FUNCTION_BLOCK "fb_517_alarm"
TITLE =Alarm-Modul (control buzzer and collective lamp)
//version!date    !author !change_segm!change_description
//-------+--------+-------+-----------+-------------------------------
// 1.0   !12.01.00!Kahle  ! ---       ! 1st version
// 1.1   !09.05.00!Kahle  ! 2         ! memo value DBD7 was wrong ->DBD17
AUTHOR : Kahle
FAMILY : PMA71
NAME : Alarm
VERSION : 1.1


VAR_INPUT
  IN_quittHorn : BOOL ;
  IN_acknowl : BOOL ;
  IN_flash : BOOL ;
END_VAR
VAR_OUTPUT
  OUT_Horn : BOOL ;
  OUT_lamp : BOOL ;
  OUT_alarm : BOOL ;
END_VAR
VAR
  Mask : ARRAY  [1 .. 5 ] OF DWORD ;
  Mask_2 : WORD ;
  memo : ARRAY  [1 .. 5 ] OF DWORD ;
  memo_2 : WORD ;
  horn_memo : BOOL ;
  alarm_memo : BOOL ;
END_VAR
VAR_TEMP
  relAlarm : ARRAY  [1 .. 5 ] OF DWORD ;
  relAlarm_2 : WORD ;
  alarmAvail : ARRAY  [1 .. 6 ] OF BOOL ;
END_VAR
BEGIN
NETWORK
TITLE =Geneate a collective alarm for alarm byte 1..4

      L     DB101.DBD   13;
      L     #Mask[1]; //release mask
      UD    ; //released alarms
      T     #relAlarm[1];
      L     #memo[1];
      XOD   ; //changed alarms
      L     #relAlarm[1];
      UD    ; //new alarms

      L     0;
      <>D   ; //if exist new alarms, set horn and flash lamp
      S     #horn_memo;
      S     #alarm_memo;
      L     DB101.DBD   13;
      T     #memo[1]; //store the actual alarms

      L     0;
      <>D   ;
      =     #alarmAvail[1]; //at least an alarm

NETWORK
TITLE =Geneate a collective alarm for alarm byte 5..8

      L     DB101.DBD   17;
      L     #Mask[2]; //release mask
      UD    ; //released alarms
      T     #relAlarm[2];
      L     #memo[2];
      XOD   ; //changed alarms
      L     #relAlarm[2];
      UD    ; //new alarms

      L     0;
      <>D   ; //if exist new alarms, set horn and flash lamp
      S     #horn_memo;
      S     #alarm_memo;
      L     DB101.DBD   17;
      T     #memo[2]; //store the actual alarms

      L     0;
      <>D   ;
      =     #alarmAvail[2]; //at least an alarm

NETWORK
TITLE =Geneate a collective alarm for alarm byte 9..12

      L     DB101.DBD   21;
      L     #Mask[3]; //release mask
      UD    ; //released alarms
      T     #relAlarm[3];
      L     #memo[3];
      XOD   ; //changed alarms
      L     #relAlarm[3];
      UD    ; //new alarms

      L     0;
      <>D   ; //if exist new alarms, set horn and flash lamp
      S     #horn_memo;
      S     #alarm_memo;
      L     DB101.DBD   21;
      T     #memo[3]; //store the actual alarms

      L     0;
      <>D   ;
      =     #alarmAvail[3]; //at least an alarm

NETWORK
TITLE =Geneate a collective alarm for alarm byte 13..16

      L     DB101.DBD   25;
      L     #Mask[4]; //release mask
      UD    ; //released alarms
      T     #relAlarm[4];
      L     #memo[4];
      XOD   ; //changed alarms
      L     #relAlarm[4];
      UD    ; //new alarms

      L     0;
      <>D   ; //if exist new alarms, set horn and flash lamp
      S     #horn_memo;
      S     #alarm_memo;
      L     DB101.DBD   25;
      T     #memo[4]; //store the actual alarms

      L     0;
      <>D   ;
      =     #alarmAvail[4]; //at least an alarm

NETWORK
TITLE =Geneate a collective alarm for alarm byte 17..20

      L     DB101.DBD   29;
      L     #Mask[5]; //release mask
      UD    ; //released alarms
      T     #relAlarm[5];
      L     #memo[5];
      XOD   ; //changed alarms
      L     #relAlarm[5];
      UD    ; //new alarms

      L     0;
      <>D   ; //if exist new alarms, set horn and flash lamp
      S     #horn_memo;
      S     #alarm_memo;
      L     DB101.DBD   29;
      T     #memo[5]; //store the actual alarms

      L     0;
      <>D   ;
      =     #alarmAvail[5]; //at least an alarm

NETWORK
TITLE =Geneate a collective alarm for alarm byte 21..22

      L     DB101.DBW   33;
      L     #Mask_2; //release mask
      UW    ; //released alarms
      T     #relAlarm_2;
      L     #memo_2;
      XOW   ; //changed alarms
      L     #relAlarm_2;
      UW    ; //new alarms

      L     0;
      <>I   ; //if exist new alarms, set horn and flash lamp
      S     #horn_memo;
      S     #alarm_memo;
      L     DB101.DBW   33;
      T     #memo_2; //store the actual alarms


      L     0;
      <>D   ;
      =     #alarmAvail[6]; //at least an alarm

NETWORK
TITLE =Set Horn and Lamp and quitt

      U     #IN_quittHorn;
      R     #horn_memo;
      U     #IN_acknowl;
      R     #alarm_memo;

      U     #horn_memo;
      =     #OUT_Horn;

      O(    ;
      U(    ;
      O     #alarmAvail[1];
      O     #alarmAvail[2];
      O     #alarmAvail[3];
      O     #alarmAvail[4];
      O     #alarmAvail[5];
      O     #alarmAvail[6];
      =     #OUT_alarm;
      )     ;
      UN    #alarm_memo;
      )     ;
      O(    ;
      U     #alarm_memo;
      U     #IN_flash;
      )     ;
      =     #OUT_lamp;

END_FUNCTION_BLOCK

DATA_BLOCK "CollectAlarm"
TITLE =
VERSION : 0.0

"fb_517_alarm"
BEGIN
   IN_quittHorn := FALSE;
   IN_acknowl := FALSE;
   IN_flash := FALSE;
   OUT_Horn := FALSE;
   OUT_lamp := FALSE;
   OUT_alarm := FALSE;
   Mask[1] := DW#16#0;
   Mask[2] := DW#16#0;
   Mask[3] := DW#16#0;
   Mask[4] := DW#16#0;
   Mask[5] := DW#16#0;
   Mask_2 := W#16#0;
   memo[1] := DW#16#0;
   memo[2] := DW#16#0;
   memo[3] := DW#16#0;
   memo[4] := DW#16#0;
   memo[5] := DW#16#0;
   memo_2 := W#16#0;
   horn_memo := FALSE;
   alarm_memo := FALSE;
END_DATA_BLOCK

FUNCTION "fc_opt3_collectAlarm" : VOID
TITLE =collective alarm
AUTHOR : Kahle
FAMILY : PMA71
NAME : CollAlar
VERSION : 0.1


VAR_TEMP
  common_alarm : BOOL ;
END_VAR
BEGIN
NETWORK
TITLE =Alarm generate ->FC68 "fc_add_ind"
//
// Horn Stop
      CALL "fb_517_alarm" , "CollectAlarm" (
           IN_quittHorn             := "I_MMI_SR".c_rst_alm,
           IN_acknowl               := "I_MMI_SR".c_rst_alm,//"I_MMI_SR".c_rst_alm
           IN_flash                 := "clockFreq_2Hz",//clockFreq_2Hz
           OUT_Horn                 := "OUT_horn",//OUT_horn
           OUT_lamp                 := "OUT_alarm",//OUT_alarm
           OUT_alarm                := "OUT_noPMA_fail");//OUT_noPMA_fail

      UN    #common_alarm;
      =     "OUT_noPMA_fail";
END_FUNCTION

